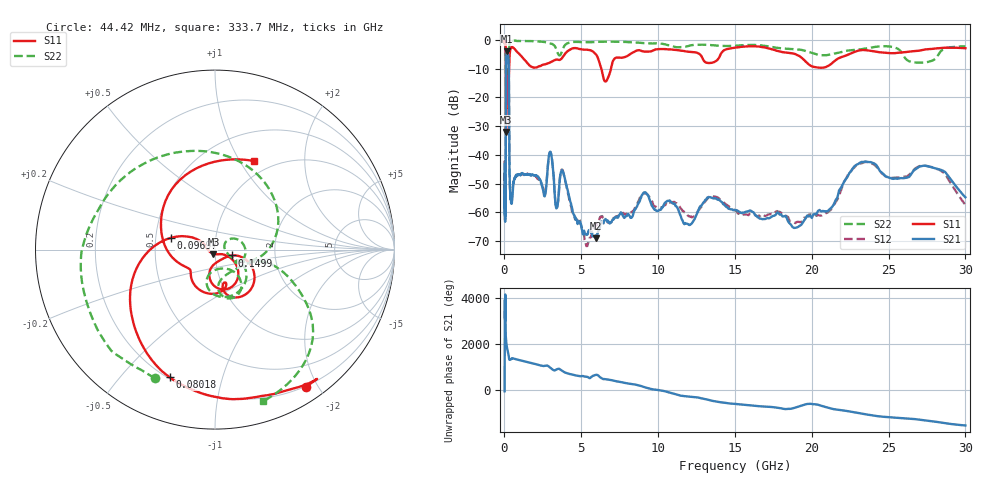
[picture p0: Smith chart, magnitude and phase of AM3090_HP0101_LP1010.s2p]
! Date/Time: Thu, Feb 28, 2019 1:59 PM
! Network Analyzer: Agilent Technologies E8364B Rev: A.07.50.67
! Sweep from 0.010 to 30.000 GHz, 1601 Points, Sweep Type: LOG
! Power Supply: 5.023 V, 0.002 A
# Hz S DB R 50
!freq MagS11 AngS11 MagS21 AngS21 MagS12 AngS12 MagS22 AngS22
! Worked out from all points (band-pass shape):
!   1601 points, 10 MHz to 30 GHz, reference 50 ohm
!   highest |S21| = -3.90 dB at 156.8 MHz (marker M1); lowest = -69.0 dB at 5.959 GHz (marker M2)
!   |S21| within 3 dB of the highest: 108.1 MHz to 271.1 MHz (163 MHz wide, 86 % of centre)
!   lowest |S11| = -32.0 dB at 105.1 MHz (marker M3), VSWR 1.05, Z = 49.1 - j2.32 ohm
!   |S11| at or under -10 dB: 95.91 MHz to 297.8 MHz (201.9 MHz wide, 103 % of centre); 6.308 GHz to 6.931 GHz (622.8 MHz wide, 9.41 % of centre)
!   |S22| runs from -25.4 to -0.2 dB; largest |S21 - S12| = 0.014
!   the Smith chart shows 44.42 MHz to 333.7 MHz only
!   S11 on the Smith chart (normalised r, x): 44.42 MHz: 0.19, -1.85; 80.18 MHz: 0.21, -0.69; 96.97 MHz: 0.60, +0.08; 149.9 MHz: 1.21, -0.08; 333.7 MHz: 0.83, +1.16
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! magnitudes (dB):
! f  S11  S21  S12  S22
! 10 MHz  -0.3  -43.3  -42.3  -0.6
! 38.04 MHz  -0.5  -60.1  -59.3  -1.6
! 44.42 MHz  -0.7  -60.0  -57.4  -2.0
! 80.18 MHz  -2.4  -49.5  -48.9  -4.7
! 96.97 MHz  -11.8  -16.1  -16.1  -11.4
! 105.1 MHz  -32.0  -8.0  -8.0  -24.6
! 120.9 MHz  -12.9  -5.2  -5.1  -16.5
! 144.7 MHz  -23.5  -4.0  -4.0  -17.6
! 149.9 MHz  -20.0  -4.0  -3.9  -17.2
! 156.8 MHz  -14.6  -3.9  -3.9  -15.4
! 274.6 MHz  -14.7  -7.4  -7.4  -16.2
! 333.7 MHz  -5.4  -47.5  -47.9  -1.1
! 550.5 MHz  -2.7  -52.2  -51.0  -0.3
! 2.084 GHz  -9.6  -47.2  -47.5  -0.5
! 2.987 GHz  -7.8  -38.9  -39.0  -1.2
! 3.385 GHz  -6.8  -58.6  -58.6  -3.4
! 3.798 GHz  -5.9  -45.7  -45.5  -3.2
! 5.959 GHz  -5.0  -69.0  -64.1  -0.7
! 7.926 GHz  -5.8  -61.3  -60.9  -0.7
! 19.22 GHz  -5.7  -64.6  -63.4  -3.4
! 23.48 GHz  -3.5  -42.3  -42.4  -3.0
! 30 GHz  -2.8  -54.7  -57.4  -2.2
